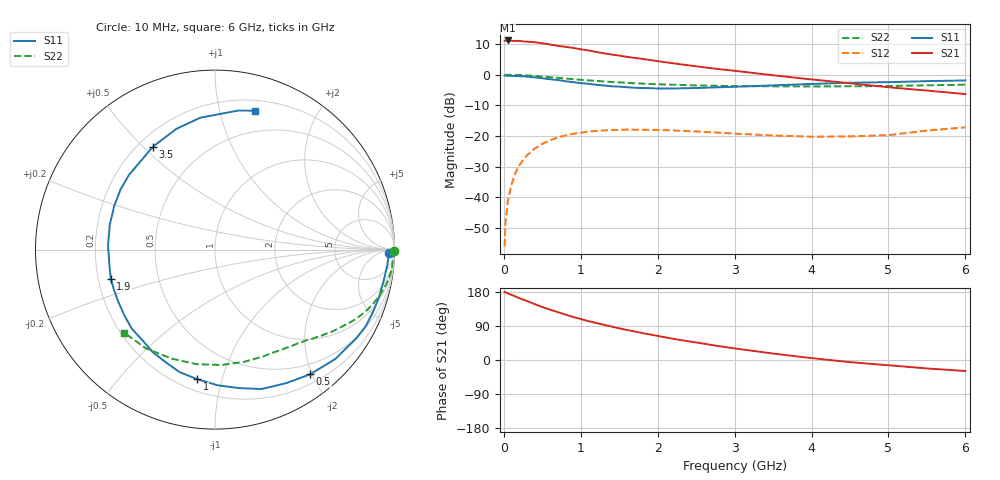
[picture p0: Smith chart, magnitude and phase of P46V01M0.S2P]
! SIEMENS Small Signal Semiconductors
! BFP182
! Si NPN RF Bipolar Junction Transistor in SOT143
! VCE = 6 V  IC = 1 mA
! Common Emitter S-Parameters:  March  1996
# GHz  S  MA  R  50
!  f  S11  S21  S12  S22
! GHz  MAG  ANG  MAG  ANG  MAG  ANG  MAG  ANG
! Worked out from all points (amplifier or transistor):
!   36 points, 10 MHz to 6 GHz, reference 50 ohm
!   highest |S21| = 11.2 dB at 50 MHz (marker M1)
!   |S21| within 3 dB of that: start of sweep to 1.033 GHz
!   unconditionally stable (mu >= 1): 2.668 GHz to end of sweep
!   at 250 MHz: K = 0.09, MSG = 19.3 dB, |S12| = -27.9 dB
!   at 1.4 GHz: K = 0.53, MSG = 12.3 dB, |S12| = -18.1 dB
!   at 6 GHz: K = 1.07, MAG = 3.8 dB, |S12| = -17.2 dB
!   S11 on the Smith chart (normalised r, x): 10 MHz: 45, -26; 500 MHz: 0.34, -1.98; 1 GHz: 0.27, -0.83; 1.9 GHz: 0.25, -0.13; 3.5 GHz: 0.26, +0.54; 6 GHz: 0.29, +1.29
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0.01  0.967 -1.1  3.575 179.5  0.0016 90.2  0.9978 -0.4
0.02  0.9678 -2.3  3.578 178.9  0.0036 88.4  0.9927 -0.7
0.05  0.9639 -5.3  3.616 175.9  0.0085 88.4  0.9965 -1.9
0.1  0.9552 -10.8  3.573 171.8  0.0162 82.9  0.9919 -4.0
0.2  0.9466 -21.6  3.558 163.4  0.0331 76.2  0.9865 -7.9
0.4  0.9057 -42.3  3.392 147.4  0.0621 63.9  0.9547 -15.2
0.5  0.8741 -52.6  3.255 139.7  0.0745 57.7  0.933 -18.6
0.6  0.8434 -61.9  3.111 133.0  0.0853 52.3  0.9116 -21.7
0.8  0.7826 -80.3  2.846 119.9  0.1021 42.5  0.8676 -27.0
0.9  0.756 -88.9  2.737 113.7  0.1087 38.1  0.8452 -29.3
1  0.7286 -97.9  2.595 108.1  0.113 34.0  0.8248 -31.5
1.1  0.7102 -106.2  2.49 102.6  0.1179 30.3  0.8074 -33.6
1.3  0.6675 -121.6  2.236 92.9  0.1232 23.4  0.775 -37.3
1.5  0.6395 -136.4  2.052 83.5  0.126 17.9  0.7486 -40.6
1.9  0.6032 -164.3  1.735 67.4  0.1261 9.3  0.7061 -46.9
2.2  0.5963 177.8  1.533 56.0  0.1233 4.6  0.6863 -51.5
2.8  0.624 147.4  1.231 36.4  0.1133 -0.8  0.6564 -61.7
3.5  0.6698 121.1  0.979 17.0  0.102 -1.4  0.6461 -75.5
4  0.7063 107.7  0.837 5.0  0.0975 2.8  0.6438 -86.9
4.5  0.7393 96.4  0.725 -5.7  0.0987 7.5  0.6466 -99.2
5.5  0.785 80.6  0.551 -22.3  0.1226 16.7  0.6716 -124.9
6  0.8054 73.9  0.483 -29.1  0.1387 15.7  0.6859 -137.6
